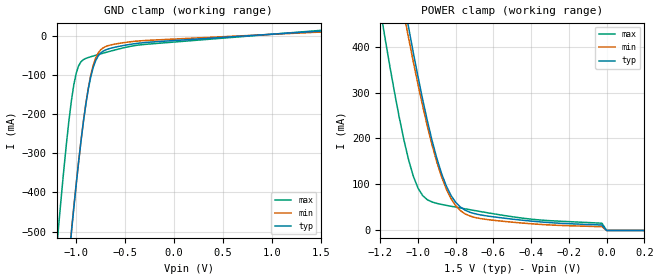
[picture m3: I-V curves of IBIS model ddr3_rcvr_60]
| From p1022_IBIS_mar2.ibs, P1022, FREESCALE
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| * P1022 DDR3 Receiver Model - 60 Ohm Termination *
[Model]   ddr3_rcvr_60
Model_type Input
Polarity   Non-Inverting
Vinl = 0.575V
Vinh = 0.925V
|   typ   min   max
C_comp   3.648330e-12   2.038670e-12   4.817820e-12
|   typ   min   max
[Voltage range]   1.5V   1.4V   1.6V
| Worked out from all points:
|   POWER clamp passes 1 mA (typ) near -0.00 V on its own axis
[GND_clamp]
| Voltage   I(typ)   I(min)   I(max)
-1.5V     -1.835A    -1.807A    -1.469A
-1.2V     -924.2mA   -913.7mA   -546.5mA
-1.175V   -851.9mA   -842.8mA   -475.7mA
-1.1V     -641.3mA   -635.7mA   -278.4mA
-1.05V    -507.8mA   -504.2mA   -169.8mA
-1V       -382.6mA   -380.5mA   -96.92mA
-925mV    -219.5mA   -217.9mA   -61.25mA
-875mV    -136.3mA   -133.3mA   -55.83mA
-825mV    -81.04mA   -75.57mA   -52.01mA
-775mV    -52.32mA   -44.69mA   -48.42mA
-700mV    -36.64mA   -28.06mA   -43.16mA
1.5V      11.5mA     9.102mA    13.35mA
[POWER_clamp]
| Table entry for 0V is set to 0.00 to avoid
| double counting with GND_clamp table
| Voltage   I(typ)   I(min)   I(max)
-1.5V     1.59A      1.496A     1.292A
-1.2V     801.1mA    756mA      480.9mA
-1.175V   738.6mA    697.3mA    418.9mA
-1.075V   498.5mA    471.9mA    197.4mA
-1.05V    441.8mA    418.6mA    153.8mA
-1V       334.4mA    317.4mA    92.1mA
-950mV    237.7mA    226mA      66.69mA
-900mV    156.5mA    148.4mA    58.9mA
-850mV    96.8mA     90.04mA    54.6mA
-750mV    44.05mA    36.06mA    47.05mA
0V        0A         0A         0A
200mV     0A         0A         0A
